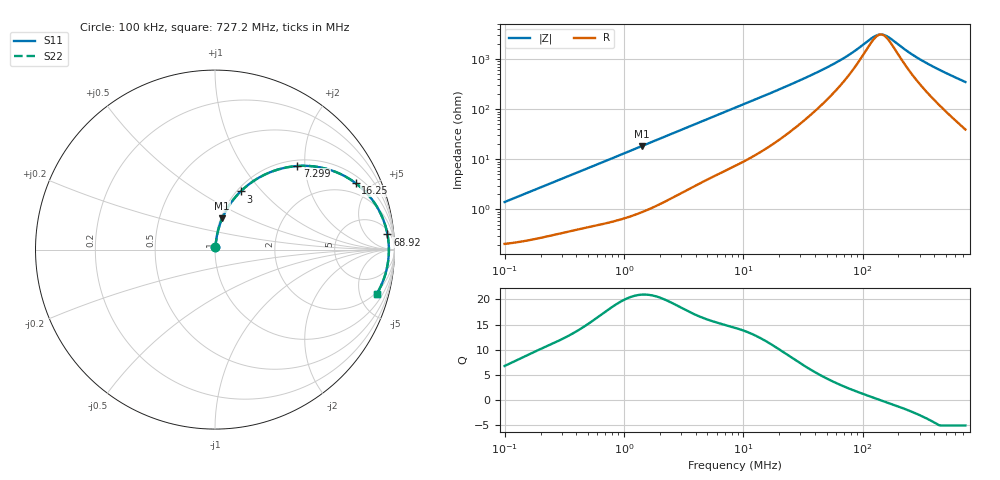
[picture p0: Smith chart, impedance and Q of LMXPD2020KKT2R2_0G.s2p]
! LMXPD2020KKT2R2_0G  S-PARAMETER MODEL  ( General Type )
! Model Generated by TAIYO YUDEN Corporation (https://www.yuden.co.jp/en/)
! Version 1.0
! TAIYO YUDEN Control No. 191023NI43SB-FBB
! Copyright(c) 2019 TAIYO YUDEN CO.,LTD. All Rights Reserved.
! Product Description (link to TY-COMPAS)
! https://ds.yuden.co.jp/TYCOMPAS/or/detail?pn=LMXPD2020KKT2R2M0G&u=M
! Products Name : Inductors
! Characteristics :
!  Inductance : 2.2 uH , SRF(min) : -Hz , DC Resistance(max) : 0.21 Ohm
!  Rated Current : Saturation :1100 mA , Temp Rise : 1100 mA (40 degC)
!  Case Size : 2.0 x 2.0 / 0.079 x 0.079 [mm/inch] , Thickness : 1 / 0.039 [mm/inch]
!  (Conditions: Temperature = 25 degC , DC Bias Current/Voltage = 0A / 0V)
! External Node Assignments :
!  1  o---GGG---o  2
! GND o---------o GND
! Frequency Range : 0.1MHz  -  727.209926MHz  [ 402 STEP ]
# MHz S RI R 50
! Freq[MHz].  S11 Real  S11 Imag  S21 Real  S21 Imag  S12 Real  S12 Imag  S22 Real  S22 Imag
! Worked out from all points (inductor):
!   401 points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, 100 kHz to 727.2 MHz, reference 50 ohm
!   read as one part in series: L = 2.21 uH near 104.5 kHz
!   highest Q = 20.9 at 1.409 MHz (marker M1), where L = 2.08 uH
!   self-resonance near 142.2 MHz
!   S11 on the Smith chart (normalised r, x): 100 kHz: 1.00, +0.03; 3 MHz: 1.04, +0.77; 7.299 MHz: 1.12, +1.82; 16.25 MHz: 1.35, +4.02; 68.92 MHz: 8, +20; 727.2 MHz: 1.79, -6.97
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0.1  0.00224 0.0139  0.9978 -0.0139  0.9978 -0.0139  0.00224 0.0139
0.443433  0.0076 0.0587  0.9924 -0.0587  0.9924 -0.0587  0.0076 0.0587
0.826312  0.0173 0.1064  0.9827 -0.1064  0.9827 -0.1064  0.0173 0.1064
1.408782  0.0407 0.1751  0.9593 -0.1751  0.9593 -0.1751  0.0407 0.1751
1.966328  0.0715 0.2343  0.9285 -0.2343  0.9285 -0.2343  0.0715 0.2343
2.999749  0.1431 0.324  0.8569 -0.324  0.8569 -0.324  0.1431 0.324
4.576292  0.2654 0.412  0.7346 -0.412  0.7346 -0.412  0.2654 0.412
7.29879  0.4581 0.4657  0.5419 -0.4657  0.5419 -0.4657  0.4581 0.4657
8.719349  0.539 0.4647  0.461 -0.4647  0.461 -0.4647  0.539 0.4647
11.64094  0.6646 0.4358  0.3354 -0.4358  0.3354 -0.4358  0.6646 0.4358
16.24801  0.7831 0.3707  0.2169 -0.3707  0.2169 -0.3707  0.7831 0.3707
24.24236  0.877 0.2763  0.123 -0.2763  0.123 -0.2763  0.877 0.2763
37.81446  0.9318 0.181  0.0682 -0.181  0.0682 -0.181  0.9318 0.181
68.91598  0.961 0.0845  0.039 -0.0845  0.039 -0.0845  0.961 0.0845
128.421  0.9688 0.011  0.0312 -0.011  0.0312 -0.011  0.9688 0.011
137.2773  0.9689 0.00381  0.0311 -0.00381  0.0311 -0.00381  0.9689 0.00381
146.7442  0.9689 -0.00339  0.0311 0.00339  0.0311 0.00339  0.9689 -0.00339
167.6818  0.9686 -0.0179  0.0314 0.0179  0.0314 0.0179  0.9686 -0.0179
239.3053  0.9655 -0.0586  0.0345 0.0586  0.0345 0.0586  0.9655 -0.0586
319.4893  0.9593 -0.0964  0.0407 0.0964  0.0407 0.0964  0.9593 -0.0964
476.6844  0.9417 -0.1604  0.0583 0.1604  0.0583 0.1604  0.9417 -0.1604
727.2099  0.9011 -0.2472  0.0989 0.2472  0.0989 0.2472  0.9011 -0.2472
